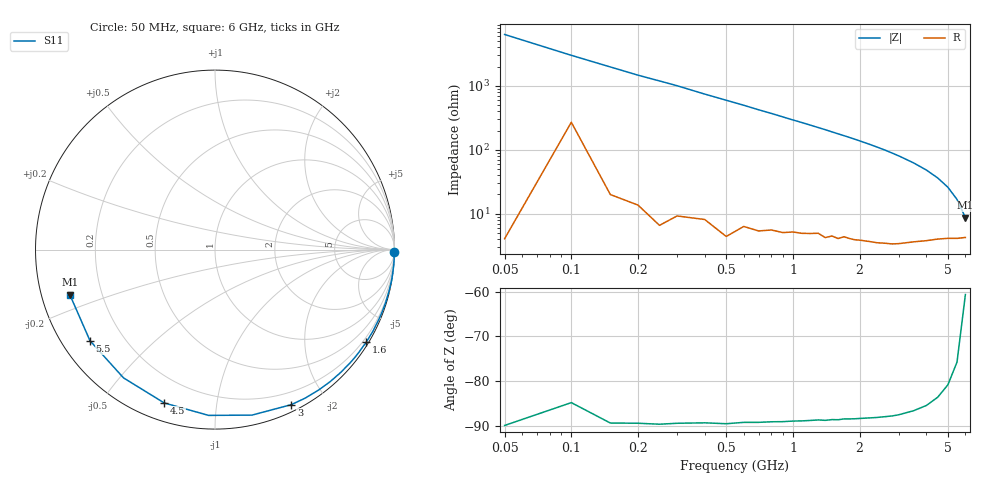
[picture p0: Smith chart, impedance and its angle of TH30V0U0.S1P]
! SIEMENS Discrete & RF Semiconductors
! BAS70
! Si Schottky Diode in SOT23
! VR = 30 V
! S-Parameters:  February  1997
# GHz  S  MA  R  50
!  f  S11
! GHz  MAG  ANG
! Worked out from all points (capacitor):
!   34 points, 50 MHz to 6 GHz, reference 50 ohm
!   read as one part to ground: C = 532 fF near 50 MHz
!   lowest |Z| = 8.66 ohm at 6 GHz (marker M1)
!   S11 on the Smith chart (normalised r, x): 50 MHz: open; 1.6 GHz: 0.08, -3.54; 3 GHz: 0.07, -1.60; 4.5 GHz: 0.08, -0.72; 5.5 GHz: 0.08, -0.32; 6 GHz: 0.08, -0.15
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0.05  1 -0.9
0.1  0.997 -1.9
0.15  0.9995 -2.9
0.25  0.9995 -4.8
0.3  0.9991 -5.7
0.4  0.9985 -7.7
0.5  0.9988 -9.6
0.7  0.997 -13.5
0.8  0.996 -15.4
1  0.9941 -19.4
1.1  0.9933 -21.3
1.2  0.992 -23.3
1.4  0.9906 -27.3
1.6  0.988 -31.5
1.8  0.9848 -35.6
1.9  0.9838 -37.7
2  0.9822 -39.9
2.2  0.9793 -44.3
2.4  0.9762 -48.9
2.6  0.9724 -53.6
2.8  0.9682 -58.7
3  0.9628 -63.8
3.5  0.9449 -77.4
4  0.9244 -92.2
4.5  0.9 -108.3
5  0.8779 -125.5
5.5  0.8619 -143.9
6  0.8468 -162.7
